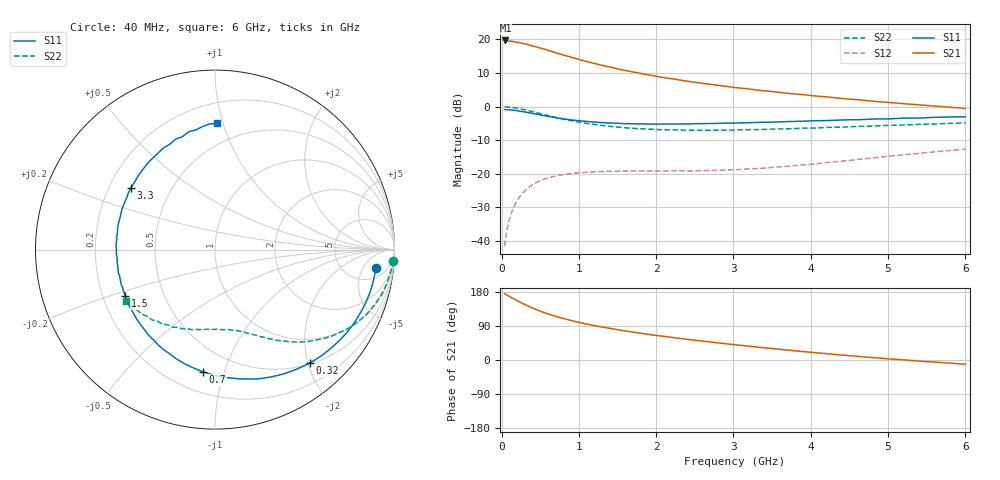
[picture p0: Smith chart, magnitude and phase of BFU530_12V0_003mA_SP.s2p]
! Filename:  P:\Prog\Test\Noise\ATS_data\Testdata_Net\03 Spar\BFU530_APG2013_40_A05_12p0V_003mA_SP_CM01_D.s2p
! Date/Time: Fri 26/Apr/2013 13:03:12
! BFU530_APG2013_40_A05_12p0V_1to25mA_SP_CM01_Bias3_R.s2p
! MDIF S-parameter v. bias file
! BFU530_APG2013_40_A05_12p0V_1to25mA_SP_CM01
! Date/time Wed Apr 24 20:41:12 2013
! VAR V_out= 12.0000
! VAR I_out= 2.9950
! VAR V_in= 0.7988
! VAR I_in= 0.0266
! Device data file deembeded for feedlines and parallel
! Original file: \03 Spar\BFU530_APG2013_40_A05_12p0V_003mA_SP_CM01_R.s2p
! Feed-files: PR047V01_250413_Feed1.s2p, PR047V01_250413_Feed2.s2p
! Parallel-file: PR047V01_250413_Par.s2p
# MHz S MA R 50
!  Freq-MHz  S11-mag  S11-arg  S21-mag  S21-arg  S12-mag  S12-arg  S22-mag  S22-arg
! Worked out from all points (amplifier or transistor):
!   98 points, 40 MHz to 6 GHz, reference 50 ohm
!   highest |S21| = 19.6 dB at 50 MHz (marker M1)
!   |S21| within 3 dB of that: start of sweep to 613.6 MHz
!   unconditionally stable (mu >= 1): 2.62 GHz to 4.579 GHz
!   at 300 MHz: K = 0.14, MSG = 21.9 dB, |S12| = -25.1 dB
!   at 1.6 GHz: K = 0.66, MSG = 15.0 dB, |S12| = -19.2 dB
!   at 6 GHz: K = 0.82, MSG = 6.1 dB, |S12| = -12.6 dB
!   S11 on the Smith chart (normalised r, x): 40 MHz: 9, -10; 320 MHz: 0.52, -2.04; 700 MHz: 0.33, -0.85; 1.5 GHz: 0.29, -0.22; 3.3 GHz: 0.29, +0.30; 6 GHz: 0.34, +0.96
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40  0.9043 -6.5  9.582 175.2  0.008415 84.9  0.9926 -3.6
50  0.9015 -8.1  9.6 173.2  0.01047 83.9  0.9938 -4.5
70  0.8992 -11.2  9.481 171.7  0.01455 82.4  0.9878 -6.5
120  0.8904 -19.5  9.395 165.7  0.02463 78.0  0.9753 -11.1
220  0.8609 -35.2  8.986 154.8  0.04303 69.4  0.9356 -19.8
320  0.823 -50.0  8.478 144.6  0.05852 61.5  0.8852 -27.7
420  0.7834 -63.5  7.881 135.7  0.07096 54.8  0.8289 -34.3
500  0.752 -73.6  7.415 129.2  0.07903 50.1  0.7859 -38.9
600  0.7151 -85.2  6.878 121.8  0.08682 45.1  0.7348 -44.0
700  0.6837 -95.6  6.329 115.3  0.09273 40.9  0.6897 -48.3
850  0.646 -109.4  5.619 106.8  0.09939 36.0  0.6325 -53.5
1050  0.6071 -125.2  4.848 97.1  0.1046 31.0  0.5736 -59.5
1200  0.5874 -135.4  4.374 90.8  0.1071 28.3  0.5408 -63.1
1500  0.5641 -152.6  3.64 80.0  0.1096 24.9  0.4957 -69.4
1750  0.5516 -164.7  3.182 72.2  0.1103 23.4  0.4706 -74.1
2050  0.5494 -176.7  2.753 63.7  0.1102 23.0  0.4538 -79.5
2450  0.5536 168.5  2.336 53.3  0.1106 24.1  0.4444 -86.9
3100  0.5712 149.2  1.874 38.6  0.1165 29.1  0.4503 -98.1
3300  0.5807 143.8  1.765 34.3  0.1198 30.7  0.4547 -101.7
4100  0.616 124.5  1.421 18.6  0.1424 35.9  0.4815 -116.1
5200  0.6734 102.5  1.104 0.5  0.1919 35.9  0.5302 -135.7
6000  0.7029 88.9  0.9404 -11.2  0.2331 31.4  0.5716 -149.7
